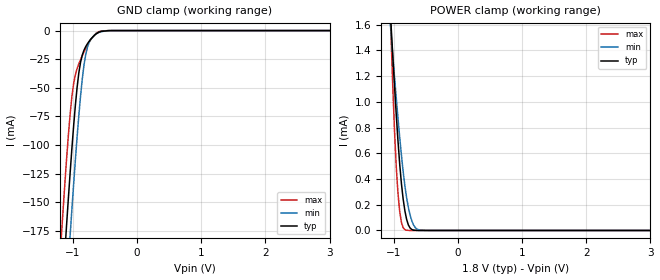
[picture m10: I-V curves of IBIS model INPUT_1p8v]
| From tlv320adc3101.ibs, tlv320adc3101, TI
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|   INPUT_1p8v
[Model]   INPUT_1p8v
Model_type   Input
Vinl = 0.54
Vinh = 1.26
|   typ   min   max
C_comp   1.022pF   1.010pF   1.056pF
[Voltage Range]   1.8   1.7   1.9
[Temperature Range]   27   85   -40
[Power Clamp Reference]   1.8   1.7   1.9
[GND Clamp Reference]   -0   -0   -0
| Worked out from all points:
|   GND clamp passes 1 mA (typ) near -0.57 V on its own axis
|   POWER clamp passes 1 mA (typ) near -0.97 V on its own axis
[GND Clamp]
|   Voltage   I(typ)   I(min)   I(max)
-1.8V     -825.6mA   -883mA     -764.7mA
-1.179V   -239mA     -296.9mA   -177.9mA
-1.125V   -191.5mA   -248.7mA   -132.3mA
-1.098V   -168.4mA   -225mA     -110.8mA
-1.044V   -124mA     -178.6mA   -72.76mA
-990mV    -83.39mA   -134.3mA   -46.34mA
-936mV    -49.76mA   -93.15mA   -33.3mA
-882mV    -27.71mA   -57.21mA   -25.42mA
-828mV    -17.09mA   -30.03mA   -18.69mA
-747mV    -9.242mA   -10.25mA   -9.988mA
-612mV    -1.906mA   -2.052mA   -1.341mA
3.573V    0A         0A         0A
[POWER Clamp]
|   Voltage   I(typ)   I(min)   I(max)
-1.8V     9.273mA    6.791mA    15.12mA
-1.071V   1.849mA    1.709mA    1.926mA
-1.044V   1.6mA      1.534mA    1.51mA
-990mV    1.125mA    1.196mA    779.6uA
-963mV    903.7uA    1.032mA    498.3uA
-936mV    699uA      875uA      290.4uA
-882mV    364.6uA    585uA      62.55uA
-828mV    152.7uA    346.9uA    6.681uA
-774mV    43.17uA    179.2uA    559.8nA
-720mV    7.819uA    74.67uA    39.63nA
-585mV    57.34nA    2.276uA    0A
3.573V    0A         0A         0A
